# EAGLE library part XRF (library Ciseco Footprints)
XRF Wireless UART Serial Data Module. www.ciseco.co.uk
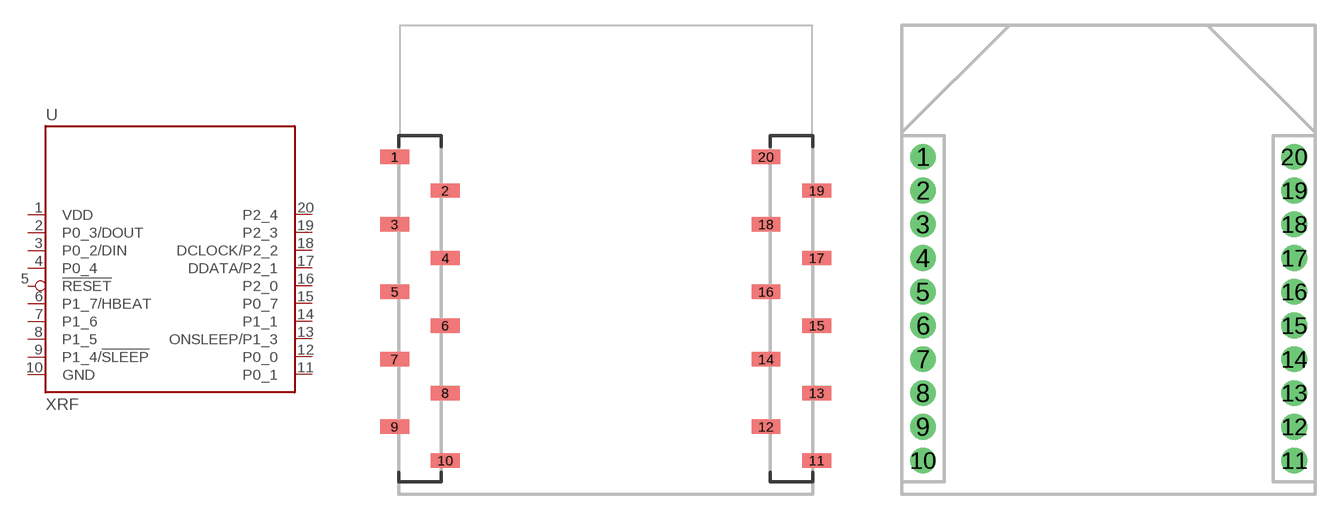
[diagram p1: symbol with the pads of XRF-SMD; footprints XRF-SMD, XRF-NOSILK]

Designator prefix U

## XRF-SMD  [XRF-SMD]
1  VDD  pwr
2  P0_3/DOUT  out
3  P0_2/DIN  in
4  P0_4
5  !RESET  in
6  P1_7/HBEAT
7  P1_6
8  P1_5
9  P1_4/!SLEEP
10  GND  pwr
11  P0_1
12  P0_0
13  ONSLEEP/P1_3
14  P1_1
15  P0_7
16  P2_0  in
17  DDATA/P2_1
18  DCLOCK/P2_2
19  P2_3
20  P2_4

## XRF-NOSILK  [XRF-NOSILK]
Pads as for XRF-SMD

## XRF-LITTLE-SILK  [XRF-LITTLE-SILK]
Pads as for XRF-SMD

## XRF-NOSLIK-LOCK-PINS  [XRF-NOSILK-LOCK-PINS]
Pads as for XRF-SMD

## XRF-NOSILK-LOCK-SOCKET  [XRF-NOSILK-LOCK-SOCKET]
Pads as for XRF-SMD

## XRF-SMD-LITTLE-SILK  [XRF-SMD-LITTLE-SLIK]
Pads as for XRF-SMD

## XRF  [XRF]
Pads as for XRF-SMD

## Footprint XRF-SMD (pad centres in mm)
smd 1.7 x 0.85: 1 -12.5,20; 2 -9.5,18; 3 -12.5,16; 4 -9.5,14; 5 -12.5,12; 6 -9.5,10; 7 -12.5,8; 8 -9.5,6; 9 -12.5,4; 10 -9.5,2; 11 12.5,2; 12 9.5,4; 13 12.5,6; 14 9.5,8; 15 12.5,10; 16 9.5,12; 17 12.5,14; 18 9.5,16; 19 12.5,18; 20 9.5,20

## Footprint XRF-NOSILK (pad centres in mm)
drill 0.8 pad 1.524: 1 -11,20; 2 -11,18; 3 -11,16; 4 -11,14; 5 -11,12; 6 -11,10; 7 -11,8; 8 -11,6; 9 -11,4; 10 -11,2; 11 11,2; 12 11,4; 13 11,6; 14 11,8; 15 11,10; 16 11,12; 17 11,14; 18 11,16; 19 11,18; 20 11,20

## Footprint XRF-LITTLE-SILK (pad centres in mm)
drill 0.8 pad 1.524: 1 -11,20; 2 -11,18; 3 -11,16; 4 -11,14; 5 -11,12; 6 -11,10; 7 -11,8; 8 -11,6; 9 -11,4; 10 -11,2; 11 11,2; 12 11,4; 13 11,6; 14 11,8; 15 11,10; 16 11,12; 17 11,14; 18 11,16; 19 11,18; 20 11,20

## Footprint XRF-NOSILK-LOCK-PINS (pad centres in mm)
As use for the XRF v2.1 PCB
drill 0.737 pad 1.524: 1 -11.095,20; 2 -10.905,18; 3 -11.095,16; 4 -10.905,14; 5 -11.095,12; 6 -10.905,10; 7 -11.095,8; 8 -10.905,6; 9 -11.095,4; 10 -10.905,2; 11 11.095,2; 12 10.905,4; 13 11.095,6; 14 10.905,8; 15 11.095,10; 16 10.905,12; 17 11.095,14; 18 10.905,16; 19 11.095,18; 20 10.905,20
